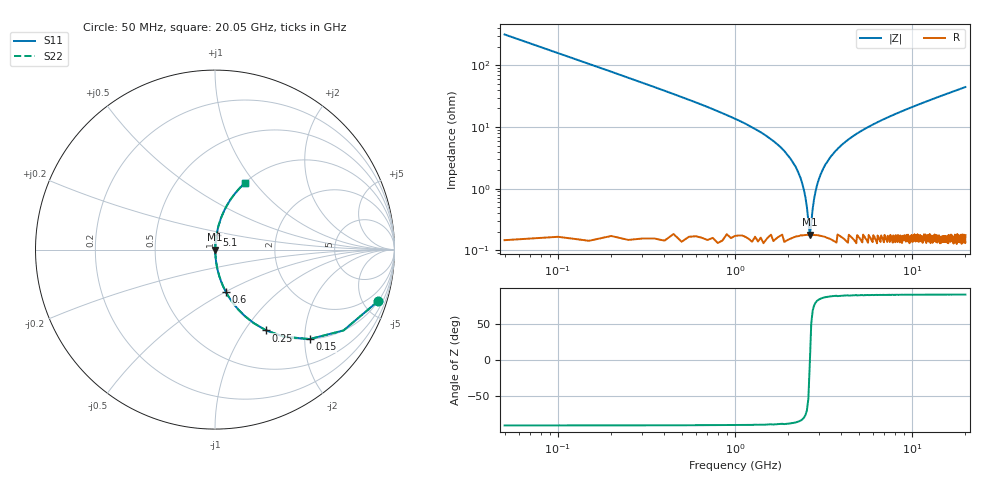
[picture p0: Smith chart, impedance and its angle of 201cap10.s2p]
! AVX Thin Film Operation		Date: May 2007
! Description: Accu-P® Series, Thin Film, SMD, RF Capacitor
! Part Number: 0201ZK100FBS
! 50 MHz  -  20.05 GHz
! Serial Measurements
# MHZ S MA R 50
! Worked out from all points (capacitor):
!   401 points, 50 MHz to 20.05 GHz, reference 50 ohm
!   read as one part in series: C = 10 pF near 150 MHz
!   lowest |Z| = 178 mohm at 2.65 GHz (marker M1)
!   series resonance near 2.653 GHz, so ESL is about 360 pH
!   S11 on the Smith chart (normalised r, x): 50 MHz: 1.00, -6.36; 150 MHz: 1.00, -2.11; 250 MHz: 1.00, -1.26; 600 MHz: 1.00, -0.50; 5.1 GHz: 1.00, +0.17; 20.05 GHz: 1.00, +0.89
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50  0.954 -17.4  0.3 72.5  0.3 72.5  0.954 -17.4
150  0.726 -43.4  0.687 46.6  0.687 46.6  0.726 -43.4
250  0.533 -57.6  0.845 32.2  0.845 32.2  0.533 -57.6
400  0.362 -68.6  0.931 21.2  0.931 21.2  0.362 -68.6
600  0.244 -75.5  0.968 14.1  0.968 14.1  0.244 -75.5
1050  0.127 -82.0  0.99 7.3  0.99 7.3  0.127 -82.0
1800  0.048 -85.4  0.997 2.7  0.997 2.7  0.048 -85.4
2150  0.025 -85.1  0.998 1.5  0.998 1.5  0.025 -85.1
2400  0.012 -82.0  0.998 0.7  0.998 0.7  0.012 -82.0
2550  0.004974 -71.6  0.998 0.3  0.998 0.3  0.004974 -71.6
2650  0.001552 -4.3  0.998 0.0  0.998 0.0  0.001552 -4.3
2750  0.004591 70.1  0.998 -0.2  0.998 -0.2  0.004591 70.1
2850  0.008746 79.3  0.998 -0.5  0.998 -0.5  0.008746 79.3
3000  0.015 83.2  0.998 -0.8  0.998 -0.8  0.015 83.2
3400  0.03 85.3  0.998 -1.7  0.998 -1.7  0.03 85.3
4050  0.052 85.3  0.997 -3.0  0.997 -3.0  0.052 85.3
5100  0.084 84.1  0.995 -4.8  0.995 -4.8  0.084 84.1
6750  0.128 82.0  0.99 -7.3  0.99 -7.3  0.128 82.0
10050  0.207 77.7  0.977 -11.9  0.977 -11.9  0.207 77.7
13400  0.279 73.5  0.959 -16.2  0.959 -16.2  0.279 73.5
16750  0.346 69.5  0.937 -20.2  0.937 -20.2  0.346 69.5
20050  0.406 65.8  0.912 -24.0  0.912 -24.0  0.406 65.8
